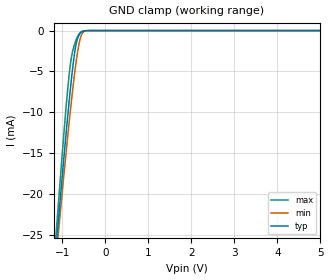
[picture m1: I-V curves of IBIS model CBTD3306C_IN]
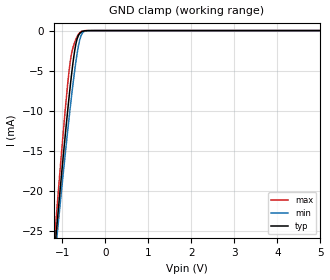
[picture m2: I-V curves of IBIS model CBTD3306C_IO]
| TEXAS INSTRUMENTS INCORPORATED
| Standard Linear and Logic Group
| IBIS Model of SN74CBTD3306C
| Dual FET Bus Switch with -2 V Undershoot Protection and Level Shifting
| This file contains package information for the following:
|  SOIC 8-pin (D) package as [Component] CBTD3306C_D
|  TSSOP 8-pin (PW) package as [Component] CBTD3306C_PW
| This device can be powered at the following Vccs:
|  5 volt Vcc
|  4 volt Vcc
| This file provides unique models under the [Model Selector] for each Vcc.
| For operation at a specific Vcc, select the appropriate model after each
| [Model Selector] keyword.
[IBIS Ver]   3.2
[Comment char]  |_char
[File Name]   sn74cbtd3306c.ibs
[File Rev]   1.1 | b_die
[Date]   June 30, 2003
[Source]   Data created from TI-SPICE simulations at TI-SLL.
[Notes]   The following is an IBIS list for the CBTD3306C.
   Please contact sllibis@ti.com with questions and
   comments concerning SLL IBIS models.
   - Power-clamp data has been deleted since there is no
   power-clamp diode in the device.
   - Non-monotonic data due to FET characteristics.
[Disclaimer] Property of Texas Instruments Incorporated.  Unauthorized
   reproduction and/or distribution is strictly prohibited.
   This product is protected under copyright law.
   Created  2003, (C) Copyright  2003, Texas Instruments
   Incorporated, All Rights Reserved
   UNLESS THERE IS A SIGNED, WRITTEN AGREEMENT TO THE
   CONTRARY, TEXAS INSTRUMENTS (TI) IS PROVIDING THE IBIS
   MODELS  AND WITHOUT ANY WARRANTY, EXPRESSED OR
   IMPLIED.  TI assumes no liability for:
   1) the accuracy of the IBIS models provided to your
   company;
   2) the proper functioning of these IBIS Models in your
   design or for any resulting applications; or
   3) infringement of patents, copyrights or intellectual
   property rights resulting from your use of these IBIS
   models.
   TI provides IBIS Models as a service to our customers.
   You and your company shall not distribute, sell or give
   these models to anyone else without prior written
   permission from TI.
   TI reserves the right to make changes to our products or
   to discontinue any semiconductor product or service
   without notice, and advises our customers to obtain the
   latest version of relevant information to verify, before
   placing orders, that the information being relied on is
   current.
   Please be aware that your receipt and use of the IBIS
   information provided shall serve as acceptance of these
   terms and conditions.  If you do not accept these terms,
   you should return or destroy the IBIS models and any
   other accompanying information immediately.
| Component CBTD3306C_D 8-pin SOIC
[Component]   CBTD3306C_D
[Manufacturer]   Texas Instruments, Inc.
[Package]
|   typ   min   max
R_pkg   2.600e-02   1.700e-02   3.500e-02
L_pkg   2.637e-09   2.180e-09   3.093e-09
C_pkg   2.690e-13   2.240e-13   3.130e-13
[Pin]   signal_name   model_name   R_pin   L_pin   C_pin
1   1NOE   CBTD3306C_IN   3.500e-02   3.093e-09   3.130e-13
2   1A   CBTD3306C_IO   1.700e-02   2.180e-09   2.240e-13
3   1B   CBTD3306C_IO   1.700e-02   2.180e-09   2.240e-13
4   GND   GND   3.500e-02   3.093e-09   3.130e-13
5   2A   CBTD3306C_IO   3.500e-02   3.093e-09   3.130e-13
6   2B   CBTD3306C_IO   1.700e-02   2.180e-09   2.240e-13
7   2NOE   CBTD3306C_IN   1.700e-02   2.180e-09   2.240e-13
8   VCC   POWER   3.500e-02   3.093e-09   3.130e-13
| Component CBTD3306C_PW 8-pin TSSOP
[Component]   CBTD3306C_PW
[Manufacturer]   Texas Instruments, Inc.
[Package]
|   typ   min   max
R_pkg   4.000e-02   3.400e-02   4.600e-02
L_pkg   2.625e-09   2.419e-09   2.861e-09
C_pkg   3.040e-13   2.860e-13   3.210e-13
[Pin]   signal_name   model_name   R_pin   L_pin   C_pin
1   1NOE   CBTD3306C_IN   4.600e-02   2.861e-09   3.210e-13
2   1A   CBTD3306C_IO   3.700e-02   2.437e-09   2.860e-13
3   1B   CBTD3306C_IO   3.400e-02   2.419e-09   2.860e-13
4   GND   GND   4.300e-02   2.784e-09   3.210e-13
5   2A   CBTD3306C_IO   4.300e-02   2.784e-09   3.210e-13
6   2B   CBTD3306C_IO   3.500e-02   2.420e-09   2.860e-13
7   2NOE   CBTD3306C_IN   3.700e-02   2.437e-09   2.860e-13
8   VCC   POWER   4.600e-02   2.860e-09   3.210e-13
[Series Switch Groups]
| Function Group States
On  1 /   | 1A->1B 1NOE LOW
On  2 /   | 2A->2B 2NOE LOW
On  1 2  /   | Enable Both
Off 1 2  /   | 1noe high, 2noe high, disable both
[Series Pin Mapping]   pin_2   model_name   function_table_group
2   3   CBTD3306C_IO_S   1
5   6   CBTD3306C_IO_S   2
[Model]   CBTD3306C_IO_S
Model_type  Series_switch
| variable   typ   min   max
C_comp   0   0   0
[Temperature Range]   40   100   -40
| Ambient temperature   25   85   -40
[Voltage range]   5   4.5   5.5
[On]
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[Off]
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| Models and submodels in the file (3): CBTD3306C_IN (Input), CBTD3306C_IO_S (Series_switch), CBTD3306C_IO (Terminator)
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| Model CBTD3306C_IN
| Model CBTD3306C_IO
| Model CBTD3306C_IO_S
[Model]   CBTD3306C_IN
Model_type  Input
Vinl=0.8
Vinh=2.0
| variable   typ   min   max
C_comp   2.48pF   1.83pF   3.30pF
[Temperature Range]   40   100   -40
| Ambient temperature   25   85   -40
[Voltage range]   5   4.5   5.5
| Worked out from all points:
|   GND clamp passes 1 mA (typ) near -0.64 V on its own axis
[GND Clamp]
| CBTD3306C_IN
|   Voltage   I(typ)   I(min)   I(max)
-5V       -300.5mA   -278.7mA   -325.7mA
-1.16V    -27.92mA   -29.02mA   -26.33mA
-1.125V   -25.71mA   -27.01mA   -23.86mA
-1.09V    -23.52mA   -25.01mA   -21.42mA
-1.06V    -21.66mA   -23.31mA   -19.35mA
-910mV    -12.7mA    -15.06mA   -9.51mA
-815mV    -7.491mA   -10.15mA   -4.404mA
-760mV    -4.802mA   -7.489mA   -2.625mA
-680mV    -1.799mA   -4.025mA   -1.206mA
-605mV    -516.4uA   -1.559mA   -393.5uA
-545mV    -167.6uA   -476uA     -102.2uA
5V        123.2pA    298.9pA    65.41pA
[Model]   CBTD3306C_IO
Model_type  Terminator
| variable   typ   min   max
C_comp   5.97pF   4.34pF   11.72pF
| C_tri-state   5.97pF   4.34pF   11.72pF
[Temperature Range]   40   100   -40
| Ambient temperature   25   85   -40
[Voltage range]   5   4.5   5.5
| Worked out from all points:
|   GND clamp passes 1 mA (typ) near -0.65 V on its own axis
[GND Clamp]
| CBTD3306C_IO
|   Voltage   I(typ)   I(min)   I(max)
-5V       -286.9mA   -267.5mA   -309.2mA
-1.19V    -28.47mA   -29.59mA   -26.88mA
-1.155V   -26.34mA   -27.64mA   -24.51mA
-1.12V    -24.23mA   -25.7mA    -22.17mA
-1.085V   -22.14mA   -23.78mA   -19.85mA
-925mV    -12.91mA   -15.26mA   -9.733mA
-815mV    -7.1mA     -9.758mA   -4.012mA
-760mV    -4.528mA   -7.197mA   -2.356mA
-675mV    -1.54mA    -3.676mA   -1.013mA
-610mV    -508.2uA   -1.614mA   -383.4uA
-545mV    -149.1uA   -450.9uA   -90.44uA
5V        473.8pA    1.464nA    157.1pA
